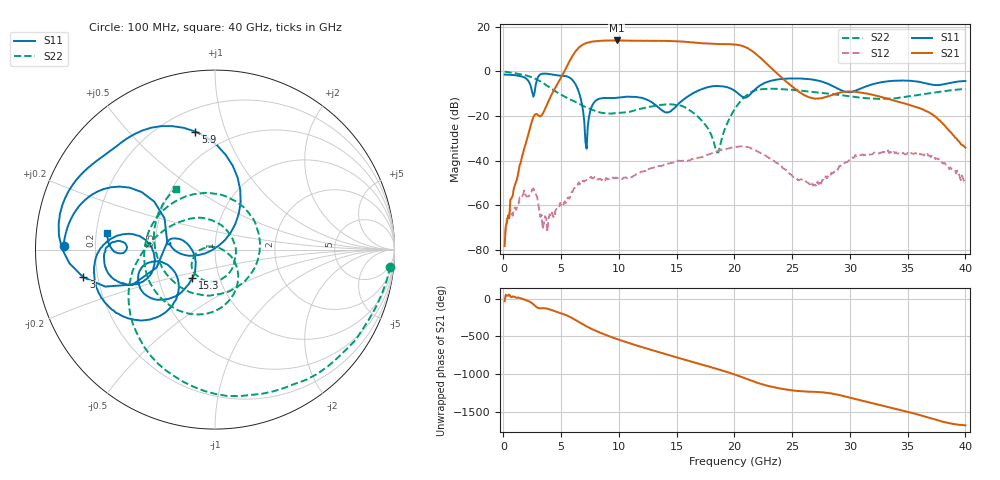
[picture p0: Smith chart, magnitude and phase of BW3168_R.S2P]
!Keysight Technologies,N5247A,US51370447,A.10.64.09
!Date: Saturday, October 09, 2021 20:39:42
!Correction: S11(Full 2 Port(1,2))
!S21(Full 2 Port(1,2))
!S12(Full 2 Port(1,2))
!S22(Full 2 Port(1,2))
!S2P File: Measurements: S11, S21, S12, S22:
# Hz S  dB  R 50
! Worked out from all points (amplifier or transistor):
!   400 points, 100 MHz to 40 GHz, reference 50 ohm
!   highest |S21| = 13.8 dB at 9.8 GHz (marker M1)
!   |S21| within 3 dB of that: 6.575 GHz to 20.96 GHz (14.39 GHz wide, 104 % of centre)
!   unconditionally stable (mu >= 1): start of sweep to end of sweep
!   at 6.7 GHz: K = 37.20, MAG = 11.8 dB, |S12| = -49.6 dB
!   at 20.1 GHz: K = 5.26, MAG = 12.7 dB, |S12| = -33.8 dB
!   at 40 GHz: K = 3667.73, MAG = -31.5 dB, |S12| = -48.6 dB
!   S11 on the Smith chart (normalised r, x): 100 MHz: 0.08, +0.01; 3 GHz: 0.14, -0.10; 5.9 GHz: 0.33, +0.79; 15.3 GHz: 0.74, -0.25; 40 GHz: 0.25, +0.07
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1e8  -1.48 178.7  -78.36 -31.9  -73.13 142.4  -0.16 -5.5
3e9  -2.50 -168.1  -19.66 -121.0  -58.84 -171.8  -3.96 -133.9
4.9e9  -1.95 135.4  -3.64 172.8  -58.98 -21.2  -10.21 160.8
5.9e9  -3.53 99.4  6.19 108.8  -54.33 -43.6  -12.89 131.8
6.8e9  -14.81 51.5  11.72 28.3  -49.79 -94.8  -15.23 102.1
7.4e9  -20.68 -161.3  12.97 -21.8  -48.39 -135.9  -16.66 82.4
8.3e9  -12.29 176.3  13.66 -85.1  -48.19 162.9  -18.36 50.7
9.8e9  -11.87 173.2  13.82 -172.6  -47.73 84.9  -18.70 1.5
1.15e10  -11.50 169.5  13.68 101.9  -46.01 19.4  -17.31 -41.0
1.24e10  -12.66 164.3  13.70 60.1  -44.01 -18.8  -16.19 -61.9
1.34e10  -16.15 168.5  13.66 14.6  -42.45 -60.0  -15.18 -84.6
1.53e10  -13.87 -128.5  13.39 -71.2  -40.18 -128.2  -15.31 -134.0
1.64e10  -9.86 -129.1  12.93 -120.0  -39.29 -157.3  -18.44 -163.3
1.76e10  -7.25 -140.2  12.48 -172.0  -37.58 169.5  -24.80 171.4
1.91e10  -6.83 -160.1  12.18 121.2  -34.97 119.0  -26.81 -2.7
2.01e10  -9.01 -169.1  11.99 70.5  -33.82 80.1  -16.35 -38.0
2.1e10  -11.74 -145.5  10.74 18.8  -33.81 39.3  -10.95 -71.6
2.21e10  -6.77 -128.7  6.74 -41.5  -36.15 -7.2  -8.21 -115.1
2.37e10  -3.68 -147.5  -0.91 -104.3  -41.15 -61.7  -7.89 -162.9
2.67e10  -3.66 -178.0  -11.98 -154.7  -49.58 -103.3  -9.23 127.7
3.34e10  -4.44 -165.7  -12.49 -2.3  -36.69 66.0  -12.29 -66.4
4e10  -4.35 171.5  -34.24 117.4  -48.58 133.2  -7.91 123.0
